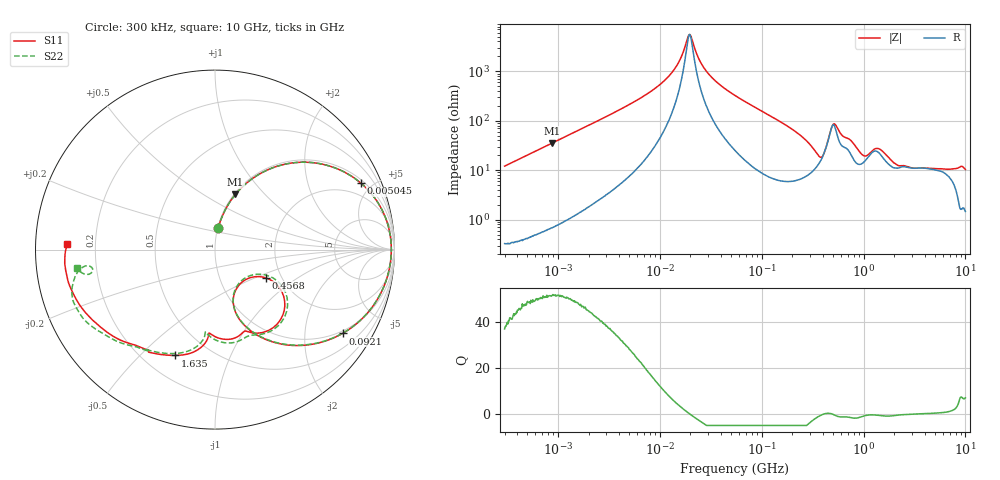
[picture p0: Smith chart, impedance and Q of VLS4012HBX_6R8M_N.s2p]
! S-Parameter Data Generated by TDK Corporation
! Copyright(C) 2023 TDK Corporation.
! All Rights Reserved.
! TDK P/N: VLS4012HBX-6R8M-N (Inductor)
! Property: L=6.8uH at 1MHz
! Size(LxWxT): 4x4x1.2mm
! Model Type: s2p (Touchstone File Format Version 1.0)
! Frequency: DC=Yes Start=0.3MHz Stop=10000MHz 802points Log-sweep
! Model Generated on June 16, 2023
! Port Assignments:
!  1 ---@@@--- 2
! Applicable Conditions:
!  Temperature = 25 degC
!  DC Bias Current = 0 A
!  Small Signal Operation
! Terms and conditions regarding TDK Simulation Models
! (1)This simulation model is being provided solely for informational purposes. Please refer to the specifications of the products in terms of detailed characteristics of such products.
! (2)In no event shall TDK Corporation of any of its subsidiaries be liable for any loss or damage arising, directly or indirectly,
!  From any information contained in this simulation model, including, but not limited to loss or damages arising from any inaccuracies, omissions or errors in connection with such information.
! (3)Any and all copyrights on this simulation model are owned by TDK Corporation.
!  Duplication or redistribution of this simulation model without prior written permission from TDK Corporation is prohibited.
! (4)This simulation model is subject to any modification or change without any prior notice.
! (5)Neither TDK Corporation nor any of its subsidiaries shall make any warranty, express or implied,
!  Including but not limited to the correctness, implied warranties of merchantability and fitness for a particular purpose with respect to this simulation models.
! (6)The use of this simulation model shall be deemed to have consented to the terms and conditions hereof.
# Hz S MA R 50
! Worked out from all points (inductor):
!   801 points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, 300 kHz to 10 GHz, reference 50 ohm
!   read as one part in series: L = 6.4 uH near 318.3 kHz
!   highest Q = 51.4 at 869.4 kHz (marker M1), where L = 6.4 uH
!   self-resonance near 19.65 MHz
!   S11 on the Smith chart (normalised r, x): 300 kHz: 1.01, +0.24; 5.045 MHz: 1.18, +4.31; 92.1 MHz: 0.92, -3.10; 456.8 MHz: 1.66, -0.59; 1.635 GHz: 0.33, -0.64; 10 GHz: 0.10, +0.02
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300000  0.1193 81.5  0.9896 -6.9  0.9896 -6.9  0.1192 81.6
869438  0.3278 69.7  0.9383 -19.2  0.9384 -19.2  0.3278 69.7
1713600  0.5617 54.5  0.8153 -34.2  0.8154 -34.2  0.5618 54.5
5044683  0.8933 24.5  0.4184 -63.5  0.4185 -63.5  0.8934 24.5
9671944  0.9667 10.5  0.1912 -75.0  0.1913 -75.0  0.9669 10.5
1.421446e7  0.9803 4.0  0.08387 -74.8  0.08388 -74.8  0.9804 4.0
1.968205e7  0.9823 -1.0  0.01772 0.2  0.01772 0.3  0.9823 -1.0
2.856806e7  0.9763 -6.8  0.09623 71.7  0.09626 71.7  0.9763 -6.8
5.477226e7  0.9362 -19.4  0.2868 66.3  0.2868 66.3  0.9363 -19.3
9.209736e7  0.8507 -33.3  0.4806 53.6  0.4807 53.6  0.8509 -33.1
1.720721e8  0.647 -54.6  0.7204 31.8  0.7205 31.8  0.6472 -54.3
3.126428e8  0.3674 -71.8  0.8523 5.6  0.8524 5.6  0.3669 -71.7
4.030213e8  0.2369 -54.0  0.8142 -10.2  0.8143 -10.2  0.23 -54.2
4.568044e8  0.3246 -29.1  0.6783 -19.3  0.6784 -19.3  0.3144 -26.7
5.105874e8  0.5138 -41.4  0.5167 -9.5  0.5168 -9.5  0.514 -38.2
5.745924e8  0.5251 -62.3  0.6205 0.5  0.6206 0.5  0.543 -59.4
9.101824e8  0.4852 -89.9  0.7602 -14.4  0.7603 -14.4  0.4892 -92.6
1.292013e9  0.525 -96.1  0.6586 -30.7  0.6587 -30.7  0.5164 -98.1
1.635219e9  0.6306 -110.8  0.6296 -35.0  0.6297 -35.0  0.6276 -112.6
1.767019e9  0.6509 -115.7  0.6245 -38.0  0.6246 -38.0  0.6491 -117.7
4.34106e9  0.8046 -154.7  0.3804 -76.8  0.3804 -76.8  0.8154 -149.3
1e10  0.825 177.9  0.2283 -111.7  0.2284 -111.8  0.7741 -172.3
